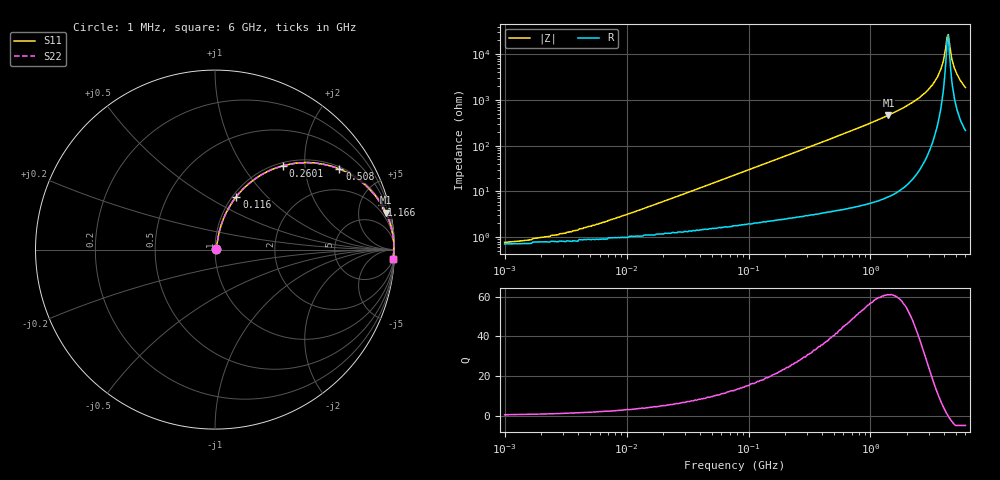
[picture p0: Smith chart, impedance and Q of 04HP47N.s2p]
# MHz S MA R 50
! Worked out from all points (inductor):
!   378 points, 1 MHz to 6 GHz, reference 50 ohm
!   read as one part in series: L = 47 nH near 10.05 MHz
!   highest Q = 61 at 1.402 GHz (marker M1), where L = 52.6 nH
!   self-resonance near 4.245 GHz
!   S11 on the Smith chart (normalised r, x): 1 MHz: 1.01, +0.01; 116 MHz: 1.04, +0.69; 260.1 MHz: 1.05, +1.54; 508 MHz: 1.08, +3.04; 1.166 GHz: 1.11, +7.43; 6 GHz: 5, -38
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1  0.007681 22.3  0.993 -0.2  0.993 -0.2  0.007681 22.3
2.349  0.01 41.0  0.992 -0.4  0.992 -0.4  0.01 41.0
4.279  0.015 55.1  0.991 -0.7  0.991 -0.7  0.015 55.1
18.312  0.055 74.9  0.987 -3.1  0.987 -3.1  0.055 74.9
78.359  0.222 72.8  0.958 -12.8  0.958 -12.8  0.222 72.8
115.999  0.319 68.0  0.929 -18.6  0.929 -18.6  0.319 68.0
260.142  0.601 51.1  0.778 -36.9  0.778 -36.9  0.601 51.1
335.312  0.695 44.2  0.698 -44.0  0.698 -44.0  0.695 44.2
507.97  0.826 32.9  0.543 -55.7  0.543 -55.7  0.826 32.9
1165.779  0.962 15.0  0.259 -74.0  0.259 -74.0  0.962 15.0
1402.133  0.974 12.1  0.21 -76.9  0.21 -76.9  0.974 12.1
1434.864  0.975 11.8  0.205 -77.3  0.205 -77.3  0.975 11.8
2439.54  0.993 5.4  0.094 -83.2  0.094 -83.2  0.993 5.4
3217.862  0.996 2.7  0.047 -84.3  0.047 -84.3  0.996 2.7
3781.976  0.997 1.2  0.021 -80.7  0.021 -80.7  0.997 1.2
3960.61  0.997 0.8  0.014 -76.1  0.014 -76.1  0.997 0.8
4244.504  0.997 0.1  0.004253 -36.4  0.004253 -36.4  0.997 0.1
4343.587  0.996 -0.1  0.003689 16.8  0.003689 16.8  0.996 -0.1
4654.933  0.996 -0.7  0.013 71.1  0.013 71.1  0.996 -0.7
4874.798  0.996 -1.1  0.02 76.5  0.02 76.5  0.996 -1.1
5470.975  0.994 -2.1  0.038 80.1  0.038 80.1  0.994 -2.1
6000  0.993 -3.0  0.053 80.4  0.053 80.4  0.993 -3.0
